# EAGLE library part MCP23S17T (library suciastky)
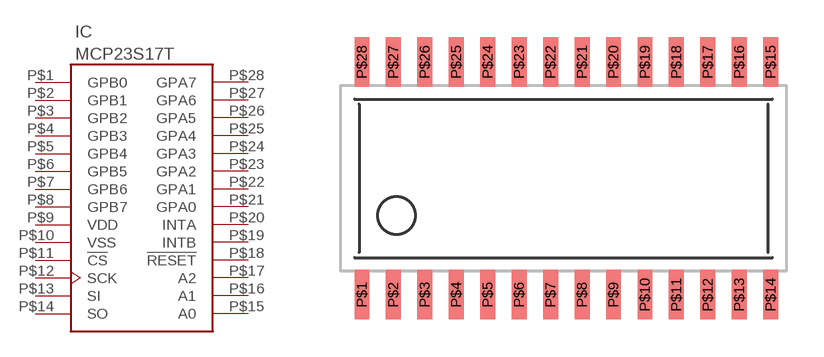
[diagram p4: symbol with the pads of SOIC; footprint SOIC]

Designator prefix IC

## MCP23S17T  [SOIC]
P$1  GPB0
P$2  GPB1
P$3  GPB2
P$4  GPB3
P$5  GPB4
P$6  GPB5
P$7  GPB6
P$8  GPB7
P$9  VDD  pwr
P$10  VSS  pwr
P$11  !CS
P$12  SCK
P$13  SI
P$14  SO
P$15  A0  in
P$16  A1  in
P$17  A2  in
P$18  !RESET
P$19  INTB  out
P$20  INTA  out
P$21  GPA0
P$22  GPA1
P$23  GPA2
P$24  GPA3
P$25  GPA4
P$26  GPA5
P$27  GPA6
P$28  GPA7

## Footprint SOIC (pad centres in mm)
smd 0.6 x 2: P$1 -8.89,-4.7; P$2 -7.62,-4.7; P$3 -6.35,-4.7; P$4 -5.08,-4.7; P$5 -3.81,-4.7; P$6 -2.54,-4.7; P$7 -1.27,-4.7; P$8 0,-4.7; P$9 1.27,-4.7; P$10 2.54,-4.7; P$11 3.81,-4.7; P$12 5.08,-4.7; P$13 6.35,-4.7; P$14 7.62,-4.7; P$15 7.62,4.7; P$16 6.35,4.7; P$17 5.08,4.7; P$18 3.81,4.7; P$19 2.54,4.7; P$20 1.27,4.7; P$21 0,4.7; P$22 -1.27,4.7; P$23 -2.54,4.7; P$24 -3.81,4.7; P$25 -5.08,4.7; P$26 -6.35,4.7; P$27 -7.62,4.7; P$28 -8.89,4.7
